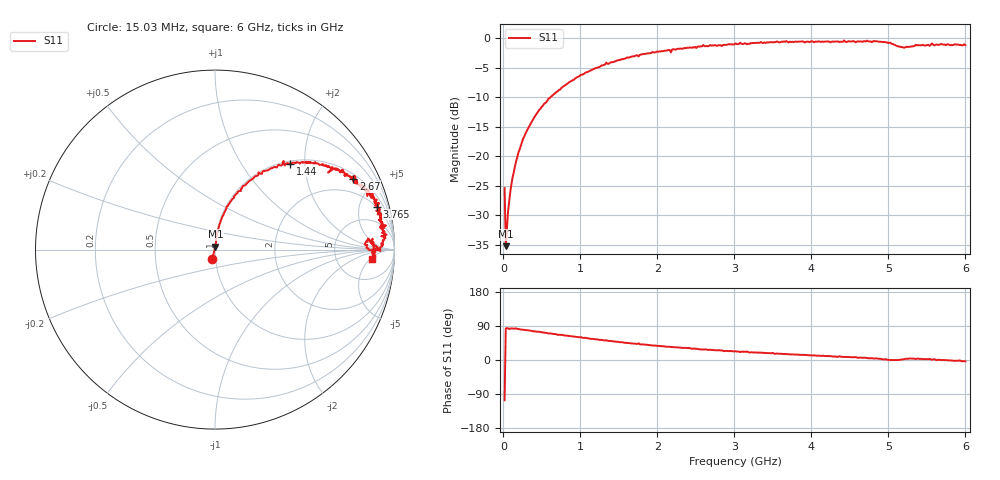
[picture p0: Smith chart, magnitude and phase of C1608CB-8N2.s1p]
!	Network	Analyzer	HP8753E.07.74:	Oct	30	2002	Serial	No.	JP38451487
!	Hewlett-Packard
!	28	Aug	2009	7:47:49
!	Frequency	S11
#	HZ	S	RI	R	50
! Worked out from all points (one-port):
!   400 points, 15.03 MHz to 6 GHz, reference 50 ohm
!   lowest |S11| = -35.2 dB at 30.03 MHz (marker M1), VSWR 1.04, Z = 50.2 + j1.73 ohm
!   |S11| at or under -10 dB: start of sweep to 607.4 MHz
!   S11 on the Smith chart (normalised r, x): 15.03 MHz: 0.97, -0.10; 1.44 GHz: 1.05, +1.69; 2.67 GHz: 1.21, +3.80; 3.765 GHz: 1.94, +7.16; 6 GHz: 13, -6
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1.502992e7  -0.0151 -0.0517
3.002985e7  0.00213 0.0172
6.00297e7  0.00399 0.034
1.050295e8  0.00689 0.0586
1.650292e8  0.00988 0.0905
2.550287e8  0.025 0.139
4.650277e8  0.065 0.24
7.650262e8  0.155 0.354
1.335023e9  0.382 0.494
1.440023e9  0.42 0.479
1.515022e9  0.448 0.481
2.265019e9  0.684 0.45
2.670017e9  0.771 0.393
3.015015e9  0.835 0.355
3.195014e9  0.848 0.298
3.495013e9  0.88 0.302
3.765011e9  0.902 0.239
4.515007e9  0.934 0.128
4.845006e9  0.946 0.0737
5.025005e9  0.922 -0.00806
5.160004e9  0.844 0.00992
5.265004e9  0.848 0.0524
5.355003e9  0.884 0.0394
5.535002e9  0.864 0.045
5.565002e9  0.907 0.0119
5.595002e9  0.875 0.0316
5.625002e9  0.89 -0.00854
6e9  0.875 -0.0511
